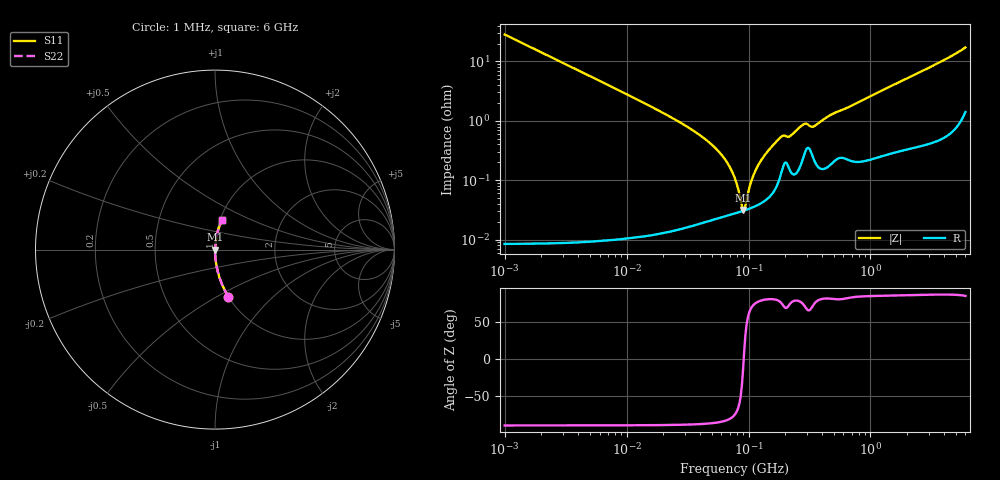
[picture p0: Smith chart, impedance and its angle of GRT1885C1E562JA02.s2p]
!Murata Part Number: GRT1885C1E562JA02
!These Parameters are Measured in Series Mode Connection
!Data Generated on Jun 19, 2026
!  o--ll--o
!Port1  Port2
!  o------o
!Operation Temp=25[degC], DC Bias Voltage=0[V]
!Freq. Start=1000[kHz] Stop=6[GHz] 401[Steps]
# Hz S RI R 50
!Freq.(Hz) S11(Real) S11(Imag) S21(Real) S21(Imag) S12(Real) S12(Imag) S22(Real) S22(Imag)
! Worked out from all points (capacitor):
!   401 points, 1 MHz to 6 GHz, reference 50 ohm
!   read as one part in series: C = 5.59 nF near 1.044 MHz
!   lowest |Z| = 31.3 mohm at 90.2 MHz (marker M1)
!   series resonance near 91.33 MHz, so ESL is about 540 pH
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1000000  0.075 -0.2633  0.925 0.2633  0.925 0.2633  0.075 -0.2633
2005636  0.0198 -0.1391  0.9802 0.1391  0.9802 0.1391  0.0198 -0.1391
4293785  0.00444 -0.0658  0.9956 0.0658  0.9956 0.0658  0.00444 -0.0658
1.843659e7  0.000342 -0.0148  0.9997 0.0148  0.9997 0.0148  0.000342 -0.0148
3.389622e7  0.000219 -0.00719  0.9998 0.00719  0.9998 0.00719  0.000219 -0.00719
5.013812e7  0.000227 -0.00393  0.9998 0.00393  0.9998 0.00393  0.000227 -0.00393
6.508975e7  0.000252 -0.00213  0.9997 0.00213  0.9997 0.00213  0.000252 -0.00213
7.745967e7  0.000276 -0.00102  0.9997 0.00102  0.9997 0.00102  0.000276 -0.00102
8.825674e7  0.000299 -0.000212  0.9997 0.000212  0.9997 0.000212  0.000299 -0.000212
9.019724e7  0.000304 -7.72e-05  0.9997 7.72e-05  0.9997 7.72e-05  0.000304 -7.72e-05
9.420718e7  0.000313 0.000193  0.9997 -0.000193  0.9997 -0.000193  0.000313 0.000193
1.050294e8  0.000341 0.000877  0.9997 -0.000877  0.9997 -0.000877  0.000341 0.000877
1.145757e8  0.000369 0.00144  0.9996 -0.00144  0.9996 -0.00144  0.000369 0.00144
1.305463e8  0.000429 0.00232  0.9996 -0.00232  0.9996 -0.00232  0.000429 0.00232
1.520136e8  0.000561 0.00346  0.9994 -0.00346  0.9994 -0.00346  0.000561 0.00346
1.848803e8  0.00131 0.0052  0.9987 -0.0052  0.9987 -0.0052  0.00131 0.0052
2.200158e8  0.00145 0.00535  0.9986 -0.00535  0.9986 -0.00535  0.00145 0.00535
2.794814e8  0.00237 0.00826  0.9976 -0.00826  0.9976 -0.00826  0.00237 0.00826
3.325952e8  0.00268 0.00742  0.9973 -0.00742  0.9973 -0.00742  0.00268 0.00742
4.919634e8  0.00215 0.0129  0.9979 -0.0129  0.9979 -0.0129  0.00215 0.0129
1.428092e9  0.00411 0.0369  0.9959 -0.0369  0.9959 -0.0369  0.00411 0.0369
6e9  0.0414 0.1624  0.9586 -0.1624  0.9586 -0.1624  0.0414 0.1624
